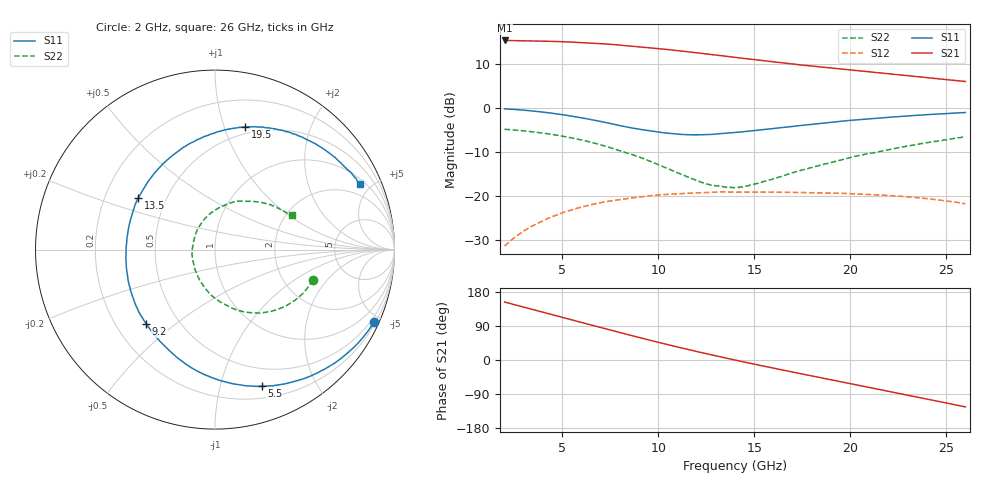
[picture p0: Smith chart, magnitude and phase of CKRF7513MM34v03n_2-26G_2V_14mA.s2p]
! CHUO DENSHI KOGYO Co.,Ltd.
! 22. July 2016
! CKRF7513MM34
! N-channel HJ-FET
! Vds = 2 V Id = 14 mA
# Hz S  MA  R 50
!	f	S11	S21	S12	S22
!	Hz	MAG	ANG	MAG	ANG	MAG	ANG	MAG	ANG
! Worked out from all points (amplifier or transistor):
!   241 points, 2 GHz to 26 GHz, reference 50 ohm
!   highest |S21| = 15.2 dB at 2 GHz (marker M1)
!   |S21| within 3 dB of that: start of sweep to 12.41 GHz
!   unconditionally stable (mu >= 1): 13.5 GHz to 19.84 GHz
!   at 6 GHz: K = 0.58, MSG = 18.6 dB, |S12| = -22.4 dB
!   at 14 GHz: K = 1.02, MAG = 14.3 dB, |S12| = -19.1 dB
!   at 26 GHz: K = 0.77, MSG = 13.8 dB, |S12| = -21.7 dB
!   lowest NFmin = 0.33 dB at 10 GHz
!   S11 on the Smith chart (normalised r, x): 2 GHz: 0.30, -4.61; 5.5 GHz: 0.31, -1.35; 9.2 GHz: 0.33, -0.40; 13.5 GHz: 0.35, +0.27; 19.5 GHz: 0.44, +1.18; 26 GHz: 1.26, +4.27
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2e9  0.9732 -24.4  5.77 152.9  0.02728 73.5  0.5716 -17.2
3e9  0.939 -37.1  5.725 139.6  0.04059 65.9  0.5484 -25.9
3.9e9  0.8976 -48.9  5.672 127.5  0.05165 58.6  0.5209 -34.1
4.8e9  0.8484 -61.2  5.603 115.3  0.06248 51.6  0.4868 -42.6
5.5e9  0.8045 -71.2  5.526 105.8  0.07018 45.8  0.456 -49.5
6e9  0.7708 -78.6  5.468 99.1  0.07543 42.0  0.4335 -54.6
6.7e9  0.7221 -89.5  5.363 89.6  0.08199 36.4  0.3978 -61.8
7.4e9  0.6725 -101.0  5.242 80.2  0.08771 30.9  0.3598 -69.5
8.1e9  0.6225 -113.0  5.086 70.9  0.09222 25.8  0.3209 -77.1
9.2e9  0.5644 -132.8  4.854 56.8  0.09945 18.2  0.2685 -90.9
1e10  0.5318 -148.3  4.672 46.7  0.1034 12.5  0.2273 -102.5
1.08e10  0.5079 -163.9  4.478 36.8  0.1061 7.3  0.1926 -115.0
1.17e10  0.495 178.6  4.258 26.0  0.1085 1.8  0.1593 -133.1
1.26e10  0.498 161.8  4.04 15.6  0.1103 -3.4  0.1373 -154.6
1.35e10  0.5153 146.2  3.832 5.3  0.1118 -9.2  0.1271 -179.3
1.4e10  0.5244 138.3  3.715 -0.2  0.1113 -11.8  0.1257 167.3
1.61e10  0.5866 110.4  3.29 -22.6  0.1111 -22.5  0.1594 120.9
1.8e10  0.6504 90.0  2.964 -42.0  0.1099 -31.5  0.2117 92.9
1.95e10  0.7037 76.1  2.744 -57.2  0.1078 -38.9  0.2554 76.5
2.2e10  0.781 55.5  2.418 -82.5  0.1021 -51.5  0.336 53.1
2.38e10  0.8311 40.8  2.217 -101.1  0.09505 -61.2  0.3959 39.0
2.6e10  0.8853 24.4  1.983 -123.7  0.08236 -73.0  0.4686 23.9
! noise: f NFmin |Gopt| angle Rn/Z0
1e+10  0.33  0.456  97.2  0.07
1.05e+10  0.35  0.442  105.1  0.06
1.1e+10  0.37  0.411  113.6  0.06
1.15e+10  0.39  0.38  124.1  0.05
1.2e+10  0.41  0.358  134.8  0.04
1.25e+10  0.43  0.337  146.9  0.04
1.3e+10  0.45  0.323  159.3  0.04
1.35e+10  0.49  0.32  172.1  0.03
1.4e+10  0.51  0.324  -174.7  0.04
1.5e+10  0.55  0.347  -153  0.04
